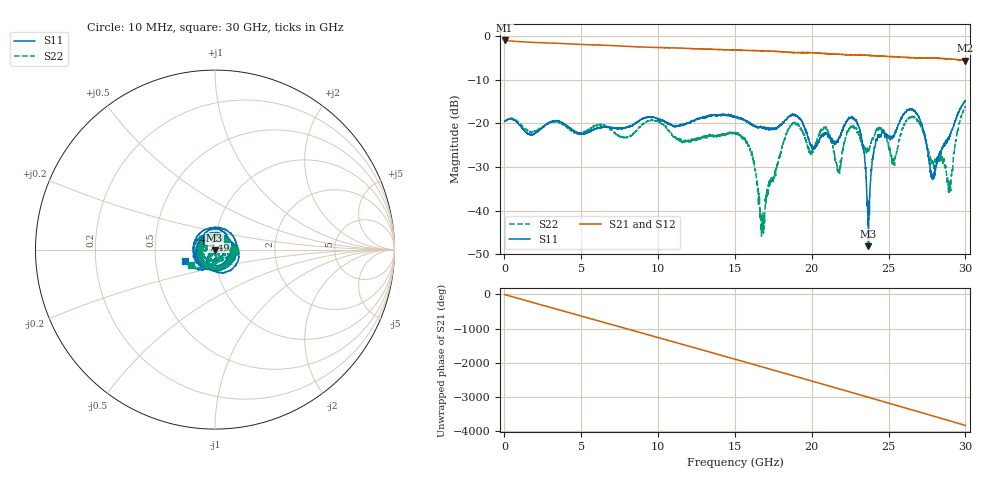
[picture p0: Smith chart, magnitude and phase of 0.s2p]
#  HZ  S  DB  R  50.00
! Rohde & Schwarz Vector Network Analyzer
! Rohde-Schwarz,ZNB40-4Port,1311601084101679,3.45
! Created: UTC 10/20/2022, 5:22:27 PM
! freq[Hz]  db:S11  ang:S11  db:S31  ang:S31  db:S13  ang:S13  db:S33  ang:S33
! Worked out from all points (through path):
!   3000 points, 10 MHz to 30 GHz, reference 50 ohm
!   highest |S21| = -1.00 dB at 10 MHz (marker M1); lowest = -5.6 dB at 30 GHz (marker M2)
!   group delay of S21, straight-line fit = 354 ps
!   lowest |S11| = -48.2 dB at 23.69 GHz (marker M3), VSWR 1.01, Z = 49.7 - j0.29 ohm
!   |S11| at or under -10 dB: start of sweep to end of sweep
!   |S22| runs from -45.9 to -16.1 dB; largest |S21 - S12| = 0.013
!   S11 on the Smith chart (normalised r, x): 10 MHz: 1.24, -0.00; 7.49 GHz: 0.87, +0.10; 30 GHz: 0.71, -0.09
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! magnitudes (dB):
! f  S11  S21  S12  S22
! 10 MHz  -19.5  -1.0  -1.0  -19.5
! 5.01 GHz  -22.3  -1.9  -1.9  -22.2
! 7.49 GHz  -21.1  -2.3  -2.3  -23.0
! 10.01 GHz  -19.1  -2.6  -2.6  -19.5
! 11.59 GHz  -20.5  -2.8  -2.8  -24.3
! 15.01 GHz  -18.5  -3.2  -3.2  -22.3
! 16.11 GHz  -20.2  -3.3  -3.3  -26.5
! 16.78 GHz  -20.9  -3.4  -3.4  -44.5
! 18.58 GHz  -18.3  -3.7  -3.7  -20.8
! 20.01 GHz  -25.0  -3.8  -3.8  -26.3
! 20.91 GHz  -22.4  -4.0  -4.0  -21.1
! 21.78 GHz  -23.1  -4.2  -4.1  -30.6
! 22.77 GHz  -19.2  -4.3  -4.3  -20.9
! 23.29 GHz  -24.3  -4.4  -4.3  -25.2
! 23.69 GHz  -48.2  -4.4  -4.4  -26.5
! 24.21 GHz  -23.6  -4.5  -4.5  -21.7
! 25.01 GHz  -23.1  -4.7  -4.6  -25.5
! 25.35 GHz  -23.1  -4.7  -4.7  -28.7
! 26.65 GHz  -17.1  -5.0  -4.9  -18.5
! 27.86 GHz  -32.4  -5.1  -5.0  -29.2
! 28.95 GHz  -23.2  -5.2  -5.2  -34.9
! 30 GHz  -14.9  -5.6  -5.6  -16.1
